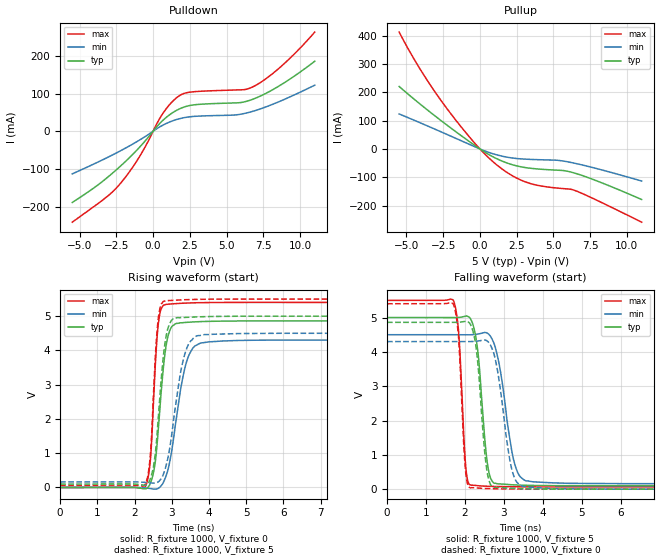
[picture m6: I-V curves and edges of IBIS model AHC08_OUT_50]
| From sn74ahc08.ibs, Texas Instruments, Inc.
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[Model]   AHC08_OUT_50
Model_type  Output
Vref =   0
Rref =   1000
Cref =   50p
Vmeas =   2.5
| variable   typ   min   max
C_comp   2.81pF   2.12pF   3.95pF
| C_pullup   3.00pF   2.15pF   3.95pF
| C_pulldown   2.63pF   2.12pF   3.31pF
[Temperature Range]   40   100   -40
| Ambient temperature   25   85   -40
[Voltage range]   5   4.5   5.5
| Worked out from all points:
|   slope of the pulldown table from 0 to 0.75 V, typ, clamps not added: 23.6 ohm
|   slope of the pullup table from 0 to 0.75 V, typ, clamps not added: 31.3 ohm
|   rising waveform, R_fixture 1000, V_fixture 0: 20-80 % time 235ps typ, 378ps min, 157ps max; typ from 0 V to 4.86 V
|   falling waveform, R_fixture 1000, V_fixture 5: 20-80 % time 212ps typ, 336ps min, 142ps max; typ from 5 V to 0.1 V
|   rising waveform, R_fixture 1000, V_fixture 5: 20-80 % time 228ps typ, 363ps min, 156ps max; typ from 0.1 V to 5 V
|   falling waveform, R_fixture 1000, V_fixture 0: 20-80 % time 206ps typ, 312ps min, 138ps max; typ from 4.86 V to 0 V
[Pulldown]
| AHC08_OUT_50
|   Voltage   I(typ)   I(min)   I(max)
-5.5V     -189.2mA   -113.2mA   -241.5mA
-3.165V   -124.5mA   -70.75mA   -174.6mA
-2.22V    -92.63mA   -51.99mA   -138.4mA
-905mV    -41.84mA   -23.06mA   -66.29mA
650mV     28.22mA    15.77mA    46.28mA
1.62V     55.79mA    31.3mA     89.43mA
2.485V    68.15mA    38.19mA    103.6mA
5.57V     75.1mA     43.06mA    109.4mA
6.775V    84.73mA    52.74mA    117.6mA
7.64V     99.74mA    63.97mA    138.2mA
8.69V     122.9mA    80.4mA     171.2mA
11V       185.8mA    122.2mA    263.1mA
[Pullup]
| AHC08_OUT_50
|   Voltage   I(typ)   I(min)   I(max)
-5.5V     220.8mA    123.8mA    412.9mA
-3.995V   155.3mA    90.82mA    275.6mA
-2.3V     86.45mA    52.58mA    146.4mA
-245mV    8.78mA     5.498mA    13.98mA
525mV     -17.33mA   -10.68mA   -27.77mA
1.285V    -37.84mA   -22.63mA   -62.15mA
2.315V    -57.24mA   -32.57mA   -97.75mA
3.345V    -67.52mA   -36.54mA   -120.7mA
5.27V     -74.95mA   -39.93mA   -138.1mA
6.32V     -83.41mA   -49mA      -144.2mA
8.125V    -116.2mA   -71.71mA   -185.4mA
11V       -178.4mA   -113.2mA   -258.6mA
[Ramp]
| AHC08_OUT_50
| variable   typ   min   max
dV/dt_r   2.94/2.45E-10   2.61/3.98E-10   3.26/1.63E-10
dV/dt_f   2.97/2.20E-10   2.64/3.52E-10   3.28/1.47E-10
R_load = 1000
[Rising Waveform]
| AHC08_OUT_50
R_fixture =   1000
C_fixture =   0
L_fixture =   0
V_fixture =   0
V_fixture_min = 0
V_fixture_max = 0
|   Time   V(typ)   V(min)   V(max)
0s        211.5pV    407.6pV    97.74pV
2.285ns   -39.65mV   -13.68mV   17.71mV
2.43ns    136.4mV    -32.38mV   852.3mV
2.555ns   728.6mV    -49.81mV   3.524V
2.64ns    1.725V     -23.8mV    4.783V
2.85ns    4.15V      349.8mV    5.346V
3.01ns    4.708V     1.146V     5.36V
3.405ns   4.821V     3.694V     5.384V
3.98ns    4.849V     4.249V     5.399V
50ns      4.861V     4.3V       5.402V
[Falling Waveform]
| AHC08_OUT_50
R_fixture =   1000
C_fixture =   0
L_fixture =   0
V_fixture =   5
V_fixture_min = 4.5
V_fixture_max = 5.5
|   Time   V(typ)   V(min)   V(max)
0s        5V         4.5V       5.5V
1.705ns   5V         4.5V       5.499V
1.84ns    5.004V     4.5V       4.569V
2.025ns   5.043V     4.498V     616.3mV
2.17ns    4.906V     4.501V     113.6mV
2.59ns    655.1mV    4.535V     84.1mV
2.85ns    153.3mV    3.808V     76.66mV
3.28ns    123.7mV    728.8mV    70.35mV
3.74ns    108.2mV    214.5mV    67.42mV
50ns      99.57mV    160.9mV    65.74mV
[Rising Waveform]
| AHC08_OUT_50
R_fixture =   1000
C_fixture =   0
L_fixture =   0
V_fixture =   5
V_fixture_min = 4.5
V_fixture_max = 5.5
|   Time   V(typ)   V(min)   V(max)
0s        99.57mV    160.9mV    65.74mV
2.285ns   67.8mV     148mV      89.49mV
2.425ns   255.3mV    135.2mV    934mV
2.545ns   875.3mV    127.3mV    3.52V
2.635ns   1.989V     162mV      4.903V
2.765ns   3.732V     357.2mV    5.422V
2.855ns   4.453V     667.9mV    5.454V
3.35ns    4.964V     3.888V     5.481V
3.885ns   4.987V     4.464V     5.495V
50ns      5V         4.5V       5.5V
[Falling Waveform]
| AHC08_OUT_50
R_fixture =   1000
C_fixture =   0
L_fixture =   0
V_fixture =   0
V_fixture_min = 0
V_fixture_max = 0
|   Time   V(typ)   V(min)   V(max)
0s        4.861V     4.3V       5.402V
1.705ns   4.86V      4.3V       5.388V
1.835ns   4.863V     4.3V       4.458V
2.015ns   4.891V     4.299V     547.6mV
2.145ns   4.793V     4.3V       34.28mV
2.56ns    577.8mV    4.327V     18.39mV
2.775ns   48.91mV    3.814V     11.96mV
3.205ns   24.87mV    574.6mV    5.151mV
3.615ns   9.917mV    60.41mV    2.225mV
50ns      -1.448nV   -11.39nV   -447.6pV
